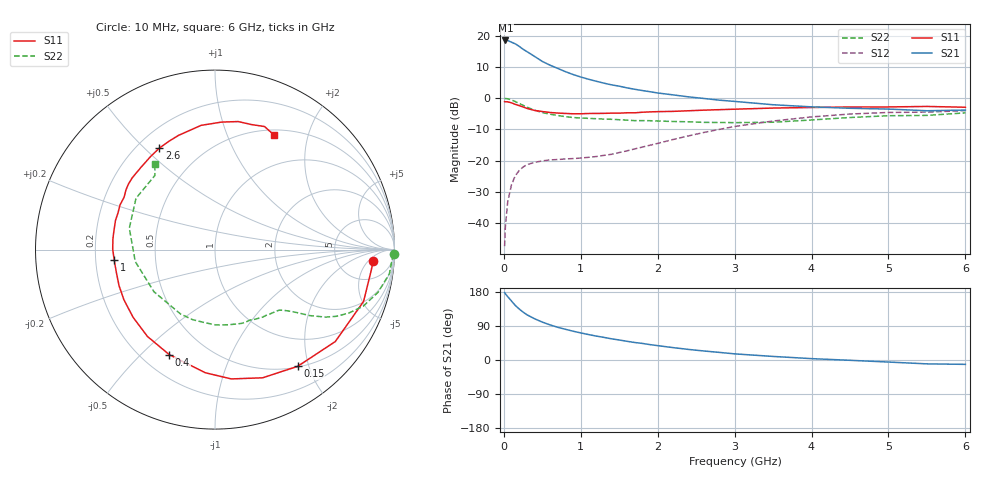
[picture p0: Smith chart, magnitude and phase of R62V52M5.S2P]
! SIEMENS Small Signal Semiconductors
! BFR193
! Si NPN RF Bipolar Junction Transistor in SOT23
! VCE = 2.5 V  IC = 2.5 mA
! Common Emitter S-Parameters:  May  1996
# GHz  S  MA  R  50
!  f  S11  S21  S12  S22
! GHz  MAG  ANG  MAG  ANG  MAG  ANG  MAG  ANG
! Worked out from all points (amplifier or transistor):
!   36 points, 10 MHz to 6 GHz, reference 50 ohm
!   highest |S21| = 18.5 dB at 20 MHz (marker M1)
!   |S21| within 3 dB of that: start of sweep to 262.8 MHz
!   unconditionally stable (mu >= 1): 1.093 GHz to 1.997 GHz
!   at 250 MHz: K = 0.27, MSG = 18.8 dB, |S12| = -22.0 dB
!   at 1.4 GHz: K = 1.10, MAG = 9.2 dB, |S12| = -17.9 dB
!   at 6 GHz: K = 0.99, MSG = 0.1 dB, |S12| = -4.0 dB
!   S11 on the Smith chart (normalised r, x): 10 MHz: 12, -7; 150 MHz: 0.51, -1.82; 400 MHz: 0.31, -0.61; 1 GHz: 0.28, -0.05; 2.6 GHz: 0.29, +0.56; 6 GHz: 0.57, +1.49
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0.01  0.8845 -4.0  8.286 177.8  0.0043 87.9  0.9965 -1.5
0.02  0.8776 -7.9  8.404 174.8  0.0088 84.5  0.9884 -3.1
0.05  0.8768 -19.2  8.373 167.3  0.0219 80.1  0.981 -7.9
0.1  0.8436 -37.4  7.873 155.5  0.0416 70.7  0.9388 -14.7
0.15  0.7969 -54.7  7.41 143.7  0.058 61.9  0.884 -20.9
0.2  0.762 -69.6  6.754 134.6  0.0698 55.5  0.8248 -25.4
0.25  0.7263 -82.8  6.085 126.4  0.0793 49.9  0.7715 -28.8
0.3  0.6882 -94.5  5.574 119.4  0.0866 46.2  0.7219 -31.4
0.4  0.6383 -113.5  4.664 108.8  0.0943 40.6  0.6425 -34.9
0.5  0.613 -127.9  3.882 100.0  0.0994 37.4  0.5904 -36.9
0.6  0.5921 -140.4  3.383 92.7  0.1031 36.0  0.5566 -38.5
0.7  0.5794 -151.1  3.005 86.3  0.1046 35.9  0.5301 -40.1
0.8  0.5713 -159.4  2.664 81.1  0.1067 36.7  0.5082 -41.7
1  0.5645 -174.0  2.186 71.5  0.1104 40.4  0.4834 -45.3
1.1  0.5699 179.7  2.016 67.2  0.1135 42.7  0.4766 -47.7
1.6  0.5848 154.7  1.466 49.4  0.144 55.4  0.4467 -60.4
2.2  0.6166 132.0  1.132 32.7  0.2188 61.0  0.4246 -80.7
2.6  0.6449 118.7  0.992 23.8  0.2834 58.6  0.4111 -97.9
3.5  0.6965 96.4  0.787 9.4  0.4322 44.0  0.4133 -145.4
4.5  0.725 79.7  0.691 -0.8  0.5587 24.3  0.492 166.0
5.5  0.7392 68.1  0.631 -10.2  0.5996 5.6  0.5318 129.0
6  0.7178 62.6  0.647 -11.5  0.6341 0.4  0.5836 125.0
